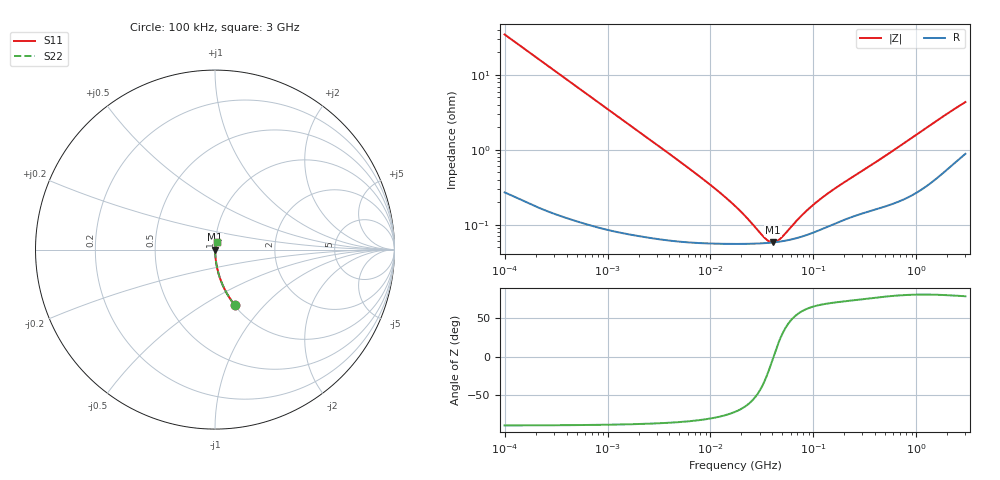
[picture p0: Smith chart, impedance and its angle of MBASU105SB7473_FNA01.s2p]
! MBASU105SB7473_FNA01  S-PARAMETER MODEL  ( Standard Model )
! Model Generated by TAIYO YUDEN Corporation (http://www.ty-top.com)
! Version 1.0
! TAIYO YUDEN Control No. 220601
! Copyright(c) 2014 TAIYO YUDEN CO.,LTD. All Rights Reserved.
! Product Description (link to TY-COMPAS)
! https://ds.yuden.co.jp/TYCOMPAS/or/detail?pn=MBASU105SB7473KFNA01&u=M
! Products Name : Multilayer Ceramic Capacitors
! Characteristics :
!  Capacitance : 0.047 [uF] , Rated Voltage : 50 [V] , TCC : X7R
!  Case Size : 1.0 x 0.5 / 0.039 x 0.02 [mm/inch] , Thickness : 0.5 / 0.02 [mm/inch]
!  (Conditions: Temperature = 25 [degC] , DC Bias Voltage = 0 [V])
! External Node Assignments :
!  1  o---| |---o  2
! GND o---------o GND
! Frequency Range : 100kHz  -  3GHz  [ 401 STEP ]
# MHZ S RI R 50
! Freq[MHz].  S11 Real  S11 Imag  S21 Real  S21 Imag  S12 Real  S12 Imag  S22 Real  S22 Imag
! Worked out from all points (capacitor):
!   401 points, 100 kHz to 3 GHz, reference 50 ohm
!   read as one part in series: C = 45.8 nF near 105.3 kHz
!   lowest |Z| = 57.9 mohm at 40.54 MHz (marker M1)
!   series resonance near 41.09 MHz, so ESL is about 330 pH
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0.1  0.1094 -0.3082  0.8906 0.3082  0.8906 0.3082  0.1094 -0.3082
0.147195  0.0546 -0.2228  0.9454 0.2228  0.9454 0.2228  0.0546 -0.2228
0.228123  0.0243 -0.1487  0.9757 0.1487  0.9757 0.1487  0.0243 -0.1487
0.344552  0.0114 -0.1  0.9886 0.1  0.9886 0.1  0.0114 -0.1
0.562235  0.0049 -0.0618  0.9951 0.0618  0.9951 0.0618  0.0049 -0.0618
1.18716  0.00168 -0.0295  0.9983 0.0295  0.9983 0.0295  0.00168 -0.0295
3.161081  0.000762 -0.0111  0.9992 0.0111  0.9992 0.0111  0.000762 -0.0111
9.331111  0.000574 -0.00361  0.9994 0.00361  0.9994 0.00361  0.000574 -0.00361
13.38544  0.00056 -0.00238  0.9994 0.00238  0.9994 0.00238  0.00056 -0.00238
17.7727  0.000555 -0.00163  0.9994 0.00163  0.9994 0.00163  0.000555 -0.00163
22.41241  0.000555 -0.00112  0.9994 0.00112  0.9994 0.00112  0.000555 -0.00112
33.85116  0.000566 -0.000338  0.9994 0.000338  0.9994 0.000338  0.000566 -0.000338
37.52708  0.000572 -0.000157  0.9994 0.000157  0.9994 0.000157  0.000572 -0.000157
40.54368  0.000578 -2.32e-05  0.9994 2.32e-05  0.9994 2.32e-05  0.000578 -2.32e-05
43.80277  0.000586 0.000111  0.9994 -0.000111  0.9994 -0.000111  0.000586 0.000111
48.55934  0.000597 0.000289  0.9994 -0.000289  0.9994 -0.000289  0.000597 0.000289
73.34282  0.000678 0.00104  0.9993 -0.00104  0.9993 -0.00104  0.000678 0.00104
97.38194  0.000775 0.00161  0.9992 -0.00161  0.9992 -0.00161  0.000775 0.00161
163.0551  0.00104 0.00288  0.999 -0.00288  0.999 -0.00288  0.00104 0.00288
547.5153  0.0019 0.0088  0.9981 -0.0088  0.9981 -0.0088  0.0019 0.0088
1838.476  0.00567 0.0274  0.9943 -0.0274  0.9943 -0.0274  0.00567 0.0274
3000  0.0105 0.0417  0.9895 -0.0417  0.9895 -0.0417  0.0105 0.0417
